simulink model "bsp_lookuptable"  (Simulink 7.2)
settings: Solver=ode45  StartTime=0.0  StopTime=20.0  RelTol=1e-3
PreLoadFcn:
  | bsp_lookuptable_ini
InitFcn:
  | bsp_lookuptable_ini
StopFcn:
  | bsp_lookuptable_plot
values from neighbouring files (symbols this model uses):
  vecin = [-10:2:10]    [bsp_lookuptable_ini.m]    (also in bsplookuptable_ini.m)
  vecout = [-5 -5 -5 -2 -2 -2 4.5 4.5 4.5 0 -1]    [bsp_lookuptable_ini.m]    (also in bsplookuptable_ini.m)
libraries: simulink x1

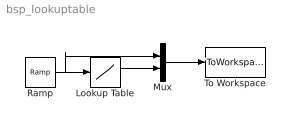
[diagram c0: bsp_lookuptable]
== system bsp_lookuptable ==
  Lookup Table : Lookup  InputValues=vecin  Table=vecout  OutDataType=sfix(16)  OutScaling=2^0
  Mux : Mux  Inputs=2
  Ramp : simulink/Sources/Ramp  SystemSampleTime=-1  slope=1  start=0  X0=-10
  To Workspace : ToWorkspace  VariableName=auslese  SampleTime=-1  SaveFormat=Array
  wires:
  Lookup Table/1 -> Mux/2
  Ramp/1 -> Lookup Table/1, Mux/1
  Mux/1 -> To Workspace/1
